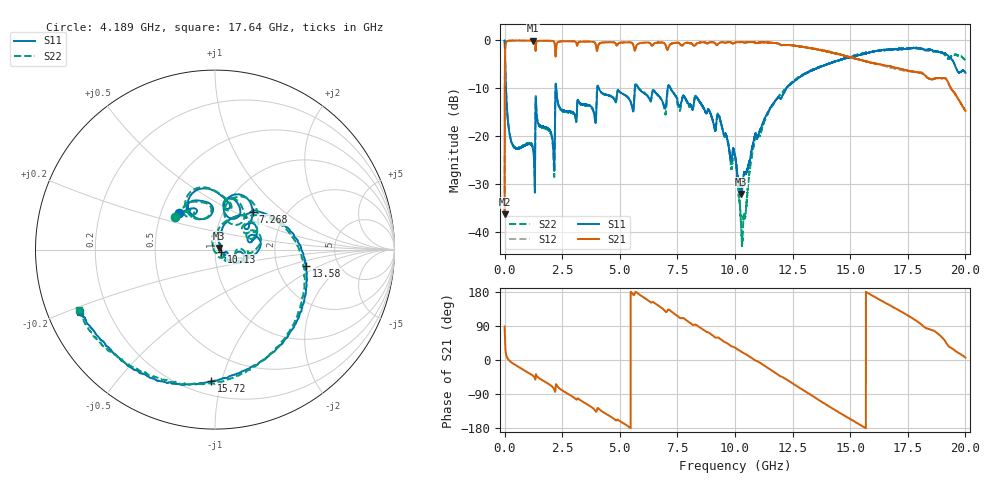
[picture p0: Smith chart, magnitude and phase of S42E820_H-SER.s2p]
!{S42E820}
!Johanson Technology Inc.
!www.johansontechnology.com
!Test Board Conditions:
!Substrate Type  RO4350B
!Substrate Thickness  50 mil
!Substrate Dk  3.66
!TL Type: GCPW
!TL Trace Width  60 mil
!TL Gap  10 mil
!Electrode orientation  Horizontal
!DUT TOPOLOGY	SERIES
!Mounting Pad LxW  14x55 mil
! Created Wed Nov 25 22:27:20 2020
# khz S ma R 50
! 2 Port Network Data from SP1.SP block
! freq  magS11  angS11  magS21  angS21  magS12  angS12  magS22  angS22
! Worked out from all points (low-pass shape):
!   20001 points, 300 kHz to 20 GHz, reference 50 ohm
!   highest |S21| = -0.03 dB at 1.228 GHz (marker M1); lowest = -36.3 dB at 300 kHz (marker M2)
!   |S21| within 3 dB of the highest: 19.61 MHz to 2.205 GHz (2.186 GHz wide, 196 % of centre); 2.22 GHz to 14.62 GHz (12.4 GHz wide, 147 % of centre)
!   lowest |S11| = -32.1 dB at 10.28 GHz (marker M3), VSWR 1.05, Z = 52.4 + j0.944 ohm
!   |S11| at or under -10 dB: 59.34 MHz to 2.21 GHz (2.15 GHz wide, 190 % of centre); 2.242 GHz to 4.021 GHz (1.778 GHz wide, 56.8 % of centre); 7.199 GHz to 12.22 GHz (5.018 GHz wide, 51.7 % of centre)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
!   |S22| runs from -43.0 to 0.0 dB; largest |S21 - S12| = 0.018
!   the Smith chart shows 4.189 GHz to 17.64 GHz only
!   S11 on the Smith chart (normalised r, x): 4.189 GHz: 0.62, +0.28; 7.268 GHz: 1.36, +0.63; 10.13 GHz: 1.07, -0.02; 13.58 GHz: 2.93, -0.72; 15.72 GHz: 0.29, -0.93; 17.64 GHz: 0.10, -0.22
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300  0.9968 -1.0  0.01525 88.2  0.01536 88.9  0.9948 -1.0
119300  0.1696 -85.2  0.984 5.3  0.9838 5.4  0.1708 -85.1
1228300  0.07477 -133.4  0.9963 -41.3  0.9951 -41.3  0.07703 -129.5
1432300  0.1402 -136.6  0.9865 -44.9  0.9863 -44.9  0.144 -131.7
2081300  0.09102 -156.6  0.9874 -71.0  0.9877 -71.1  0.08632 -157.5
2290300  0.2407 -156.0  0.948 -69.6  0.9481 -69.6  0.2372 -154.0
3334300  0.2164 158.2  0.9703 -108.0  0.9697 -108.0  0.2132 166.3
4189300  0.2876 134.7  0.9428 -133.8  0.9433 -133.8  0.2854 140.8
6667300  0.2653 58.1  0.9508 143.8  0.9478 143.8  0.2685 53.6
7268300  0.2959 45.0  0.9285 126.6  0.9283 126.5  0.2975 35.8
8585300  0.208 -11.1  0.9546 81.4  0.9542 81.4  0.205 -4.6
1.00003e7  0.06272 -27.1  0.9463 32.6  0.9467 32.6  0.06105 -46.8
1.01253e7  0.03654 -18.4  0.9573 27.4  0.9579 27.4  0.03012 -71.2
1.02763e7  0.02496 21.2  0.9607 21.8  0.9603 21.9  0.0102 -110.2
1.09023e7  0.107 65.4  0.9377 -1.9  0.9378 -1.8  0.09986 83.9
1.33343e7  0.4854 -0.9  0.8236 -93.8  0.8268 -93.6  0.4895 -6.0
1.35763e7  0.5154 -10.0  0.8036 -103.0  0.8136 -103.2  0.5175 -15.7
1.57153e7  0.7329 -91.6  0.6007 178.6  0.6045 177.9  0.7455 -92.0
1.66673e7  0.7988 -119.8  0.541 146.4  0.5276 146.5  0.8008 -125.6
1.76373e7  0.8278 -155.2  0.4736 112.6  0.4785 112.8  0.8273 -156.1
1.91933e7  0.707 139.0  0.386 42.9  0.3884 42.5  0.6596 152.9
2e7  0.4589 129.0  0.1835 6.3  0.1841 6.8  0.6138 120.2
